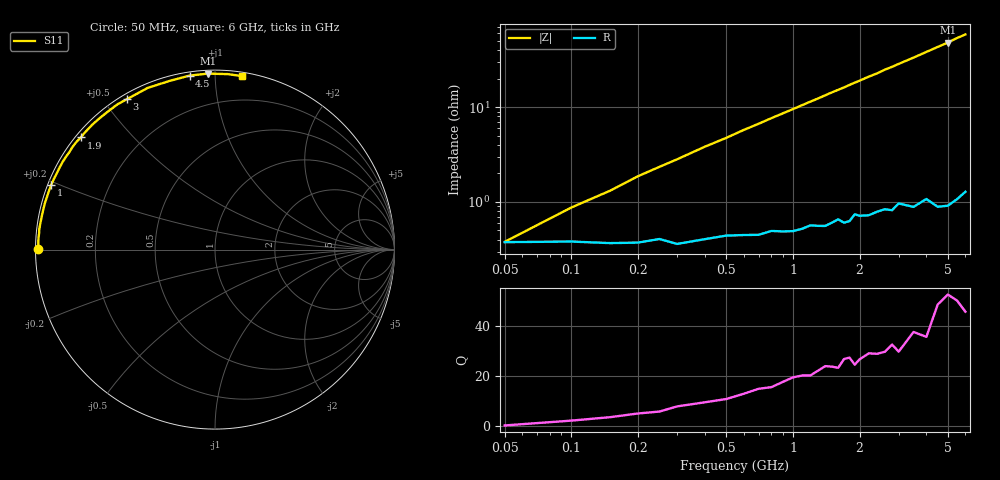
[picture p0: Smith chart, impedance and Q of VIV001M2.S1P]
! Infineon Technologies  Discrete & RF Semiconductors
! BB 804
! Si Tuning Diode in SOT23
! VR =
! S-Parameters:  July  1999
# GHz  S  MA  R  50
!  f  S11
! GHz  MAG  ANG
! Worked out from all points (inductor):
!   34 points, 50 MHz to 6 GHz, reference 50 ohm
!   read as one part to ground: L = 1.46 nH near 150 MHz
!   highest Q = 50.2 at 5 GHz (marker M1), where L = 1.53 nH
!   S11 on the Smith chart (normalised r, x): 50 MHz: 0.01, +0.00; 1 GHz: 0.01, +0.19; 1.9 GHz: 0.01, +0.36; 3 GHz: 0.02, +0.57; 4.5 GHz: 0.02, +0.86; 6 GHz: 0.03, +1.17
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0.05  0.985 179.9
0.1  0.9848 178.2
0.2  0.9852 175.8
0.3  0.9857 173.6
0.4  0.984 171.3
0.5  0.9826 169.2
0.6  0.9825 166.9
0.7  0.9825 164.8
0.8  0.9809 162.6
1  0.9812 158.4
1.3  0.9791 152.2
1.5  0.9779 148.0
1.6  0.9763 146.1
1.7  0.9784 144.2
1.8  0.9778 142.1
1.9  0.9741 140.1
2  0.9754 138.3
2.2  0.9757 134.4
2.4  0.9742 131.0
2.6  0.9735 127.1
2.8  0.9748 123.9
3  0.9714 120.4
3.5  0.9757 112.6
4  0.9733 105.1
4.5  0.9798 98.3
5  0.9812 92.3
5.5  0.9803 85.9
6  0.9786 81.0
